TYPE ST_PmlCommand :

//@details
//The FB_Base is the base function block of the .
//@usage
//The function block works like this or like that.
//also there are multiline stuff possible


STRUCT
	eMode 			: E_PmlMode;
	eState 			: E_PmlState;
	bFollow 		: BOOL;
END_STRUCT
END_TYPE
